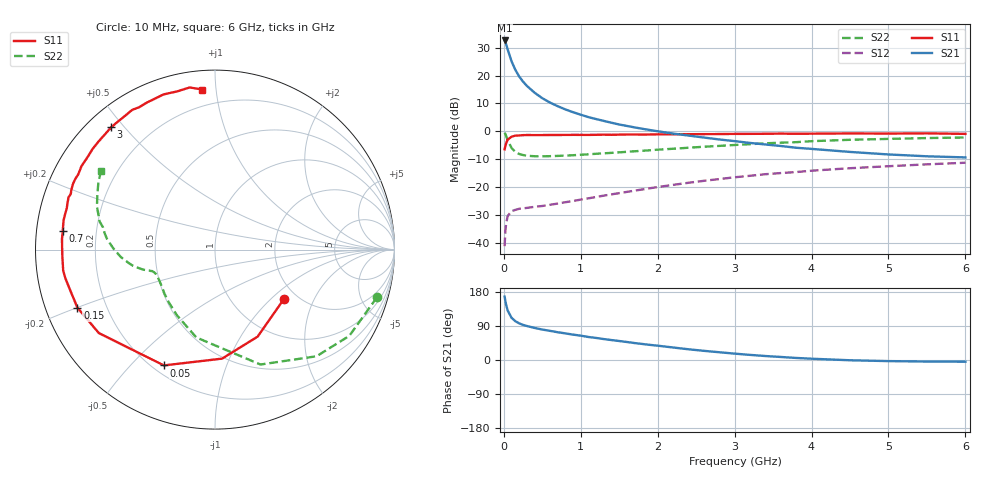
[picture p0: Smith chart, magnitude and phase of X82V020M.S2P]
! SIEMENS Small Signal Semiconductors
! BFP136W
! Si NPN RF Bipolar Junction Transistor in SOT343
! VCE = 2 V  IC = 20 mA
! Common Emitter S-Parameters:  September  1994
# GHz  S  MA  R  50
!  f  S11  S21  S12  S22
! GHz  MAG  ANG  MAG  ANG  MAG  ANG  MAG  ANG
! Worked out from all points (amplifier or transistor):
!   40 points, 10 MHz to 6 GHz, reference 50 ohm
!   highest |S21| = 32.6 dB at 10 MHz (marker M1)
!   |S21| within 3 dB of that: start of sweep to 47.49 MHz
!   unconditionally stable (mu >= 1): 823.8 MHz to 2.838 GHz; 5.993027 GHz to end of sweep
!   at 200 MHz: K = 0.34, MSG = 23.7 dB, |S12| = -27.9 dB
!   at 1.5 GHz: K = 1.16, MAG = 9.9 dB, |S12| = -22.3 dB
!   at 6 GHz: K = 1.00, MAG = 0.7 dB, |S12| = -11.3 dB
!   S11 on the Smith chart (normalised r, x): 10 MHz: 1.71, -1.21; 50 MHz: 0.24, -0.62; 150 MHz: 0.10, -0.20; 700 MHz: 0.08, +0.06; 3 GHz: 0.07, +0.46; 6 GHz: 0.10, +0.92
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0.01  0.4725 -35.6  42.64 167.4  0.0086 76.6  0.9408 -16.4
0.02  0.5399 -63.9  39.58 155.5  0.0162 67.5  0.8895 -32.7
0.03  0.6088 -86.3  36.55 145.6  0.022 58.2  0.8205 -46.4
0.05  0.7052 -113.8  29.37 130.5  0.0299 44.5  0.6887 -68.4
0.1  0.7969 -144.3  18.01 111.4  0.0366 29.6  0.5005 -102.0
0.15  0.832 -157.1  12.61 102.3  0.0386 25.3  0.4225 -120.3
0.2  0.8379 -164.3  9.577 96.6  0.0404 23.8  0.3894 -131.8
0.25  0.849 -169.2  7.757 92.6  0.0411 23.9  0.3726 -139.4
0.3  0.8538 -172.2  6.503 89.7  0.0419 24.3  0.362 -144.4
0.4  0.8513 -177.5  4.906 84.6  0.0438 26.9  0.3548 -151.1
0.5  0.8522 178.6  3.914 80.4  0.0453 29.7  0.3537 -155.2
0.6  0.8545 176.0  3.267 76.9  0.0477 32.1  0.3559 -157.5
0.7  0.8545 173.0  2.812 73.3  0.0501 35.4  0.3595 -158.9
0.9  0.8592 169.0  2.193 67.0  0.0556 39.7  0.3698 -161.1
1.1  0.8576 164.2  1.789 60.7  0.0622 43.9  0.3843 -162.3
1.5  0.8672 157.3  1.318 50.1  0.0771 49.4  0.4167 -164.6
2.2  0.8769 144.5  0.906 33.0  0.1085 51.8  0.4835 -170.8
3  0.8939 130.3  0.663 16.8  0.1485 48.4  0.5651 179.5
3.2  0.8956 126.9  0.615 13.5  0.158 47.0  0.5842 176.9
4.5  0.9109 108.3  0.424 -0.7  0.2162 35.6  0.7006 159.9
5.5  0.9143 98.9  0.354 -4.1  0.2537 27.2  0.7525 149.6
6  0.8947 94.5  0.338 -4.5  0.2713 22.6  0.7702 145.5
